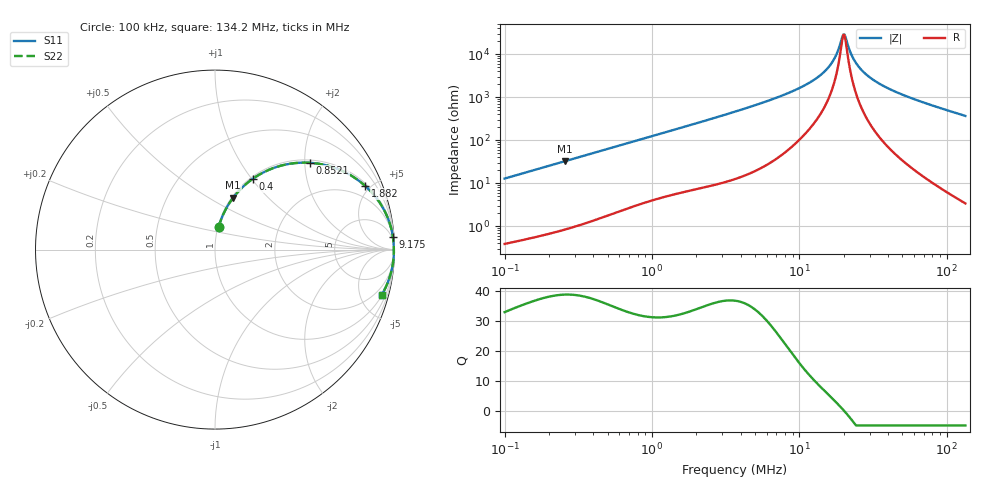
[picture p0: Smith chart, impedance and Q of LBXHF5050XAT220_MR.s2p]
! LBXHF5050XAT220_MR  S-PARAMETER MODEL  ( General Type )
! Model Generated by TAIYO YUDEN Corporation (http://www.ty-top.com)
! Version 1.0
! TAIYO YUDEN Control No. 200511NI43SB-FBB
! Copyright(c) 2020 TAIYO YUDEN CO.,LTD. All Rights Reserved.
! Product Description (link to TY-COMPAS)
! https://ds.yuden.co.jp/TYCOMPAS/or/detail?pn=LBXHF5050XAT220MMR&u=M
! Products Name : Inductors
! Characteristics :
!  Inductance : 22 uH , SRF(min) : 15 MHz , DC Resistance(max) : 0.228 Ohm
!  Rated Current : Saturation :1700 mA , Temp Rise : 800 mA
!  Case Size : 5.0 x 5.0 / 0.197 x 0.197 [mm/inch] , Thickness : 3.1 / 0.122 [mm/inch]
!  (Conditions: Temperature = 25 degC , DC Bias Current/Voltage = 0A / 0V)
! External Node Assignments :
!  1  o---GGG---o  2
! GND o---------o GND
! Frequency Range : 0.1MHz  -  134.160692MHz  [ 402 STEP ]
# MHz S RI R 50
! Freq[MHz].  S11 Real  S11 Imag  S21 Real  S21 Imag  S12 Real  S12 Imag  S22 Real  S22 Imag
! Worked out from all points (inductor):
!   401 points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, 100 kHz to 134.2 MHz, reference 50 ohm
!   read as one part in series: L = 20.4 uH near 103.7 kHz
!   highest Q = 38.9 at 255 kHz (marker M1), where L = 20.2 uH
!   self-resonance near 19.9 MHz
!   S11 on the Smith chart (normalised r, x): 100 kHz: 1.01, +0.26; 400 kHz: 1.03, +1.01; 852.1 kHz: 1.07, +2.13; 1.882 MHz: 1.14, +4.65; 9.175 MHz: 3, +28; 134.2 MHz: 1.07, -7.34
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0.1  0.02 0.1255  0.98 -0.1255  0.98 -0.1255  0.02 0.1255
0.25503  0.1013 0.2892  0.8987 -0.2892  0.8987 -0.2892  0.1013 0.2892
0.334101  0.1587 0.3526  0.8413 -0.3526  0.8413 -0.3526  0.1587 0.3526
0.400007  0.2104 0.3944  0.7896 -0.3944  0.7896 -0.3944  0.2104 0.3944
0.852057  0.5306 0.4836  0.4694 -0.4836  0.4694 -0.4836  0.5306 0.4836
1.116232  0.6536 0.4601  0.3464 -0.4601  0.3464 -0.4601  0.6536 0.4601
1.881513  0.8367 0.355  0.1633 -0.355  0.1633 -0.355  0.8367 0.355
3.729338  0.9517 0.2013  0.0483 -0.2013  0.0483 -0.2013  0.9517 0.2013
9.174552  0.9913 0.0696  0.00872 -0.0696  0.00872 -0.0696  0.9913 0.0696
12.23742  0.9944 0.0416  0.00559 -0.0416  0.00559 -0.0416  0.9944 0.0416
14.39002  0.9955 0.0274  0.00455 -0.0274  0.00455 -0.0274  0.9955 0.0274
16.32281  0.996 0.0169  0.00396 -0.0169  0.00396 -0.0169  0.996 0.0169
17.86036  0.9963 0.00952  0.00366 -0.00952  0.00366 -0.00952  0.9963 0.00952
19.54274  0.9965 0.00218  0.00345 -0.00218  0.00345 -0.00218  0.9965 0.00218
20.25926  0.9966 -0.000756  0.00339 0.000756  0.00339 0.000756  0.9966 -0.000756
20.62732  0.9966 -0.00223  0.00337 0.00223  0.00337 0.00223  0.9966 -0.00223
22.98037  0.9967 -0.0111  0.00334 0.0111  0.00334 0.0111  0.9967 -0.0111
26.06697  0.9965 -0.0217  0.00353 0.0217  0.00353 0.0217  0.9965 -0.0217
31.2091  0.9957 -0.0375  0.00428 0.0375  0.00428 0.0375  0.9957 -0.0375
40.88529  0.9933 -0.0636  0.00674 0.0636  0.00674 0.0636  0.9933 -0.0636
67.68632  0.9815 -0.1255  0.0185 0.1255  0.0185 0.1255  0.9815 -0.1255
134.1607  0.9288 -0.2525  0.0712 0.2525  0.0712 0.2525  0.9288 -0.2525
